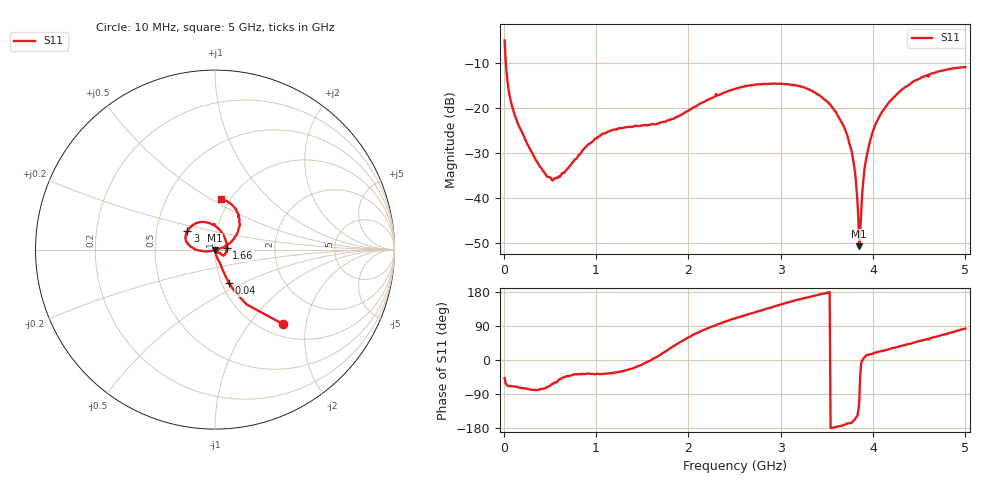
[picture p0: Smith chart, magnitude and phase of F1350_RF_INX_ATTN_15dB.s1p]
! S-parameters for RF_INX input IDT F1350 DPD Demodulator
! Date Measured:  2015-11-25  RGG
!  Port 1 = Pin 35 = RF_INX
! STATE: RF_INX selected, 15 dB attenuation (Gain = Gmax - 15 dB)
! RF Frequency:  10 MHz to 5000 MHz
! RF_INY, IF_I+, IF_I-, IF_Q+, and IF_Q- terminated
! 2300 MHz, 0 dBm signal applied to LO_IN
! Vcc = +5.00 Volts  Icc = approx 275 mA.
! NOTES:  The device was measured on a custom printed circuit evaluation board with individual 50 ohm
!  microstrip lines to the RF and LO pins. The 50 ohm microstrip lines were de-embedded using reference
!  plane extensions
! Instrument Manufacturer:  Agilent Technologies
! Instrument Model:  E5071C
! Instrument Serial Number:  MY46419053
! Instrument Firmware Rev:  A.11.31
! Frequency Re{S11} Im{S11}
# HZ  S  RI R 50.00
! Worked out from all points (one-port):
!   500 points, 10 MHz to 5 GHz, reference 50 ohm
!   lowest |S11| = -50.7 dB at 3.85 GHz (marker M1), VSWR 1.01, Z = 49.9 - j0.267 ohm
!   |S11| at or under -10 dB: 23.28 MHz to end of sweep
!   S11 on the Smith chart (normalised r, x): 10 MHz: 1.23, -1.48; 40 MHz: 1.08, -0.42; 1.66 GHz: 1.14, +0.02; 3 GHz: 0.72, +0.15; 5 GHz: 0.91, +0.56
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1e7  0.3778 -0.4147
4e7  0.0777 -0.1854
7e7  0.0455 -0.1196
1.3e8  0.0264 -0.073
3.5e8  0.00488 -0.0257
5.2e8  0.00706 -0.0143
6.4e8  0.0129 -0.0135
1e9  0.0367 -0.0278
1.26e9  0.0509 -0.0307
1.66e9  0.0657 0.00925
1.89e9  0.0573 0.0566
2.51e9  -0.0567 0.1525
3e9  -0.1546 0.1023
3.13e9  -0.1632 0.0744
3.53e9  -0.11 0.00155
3.68e9  -0.063 -0.00893
3.76e9  -0.0342 -0.0084
3.8e9  -0.0191 -0.00768
3.84e9  -0.00438 -0.00452
3.85e9  -0.00117 -0.00267
3.87e9  0.00624 -0.00116
3.9e9  0.0177 0.00155
3.92e9  0.0251 0.00472
4.01e9  0.0562 0.0184
4.17e9  0.1007 0.0547
4.38e9  0.1322 0.1188
4.63e9  0.1265 0.2043
5e9  0.0339 0.2817
